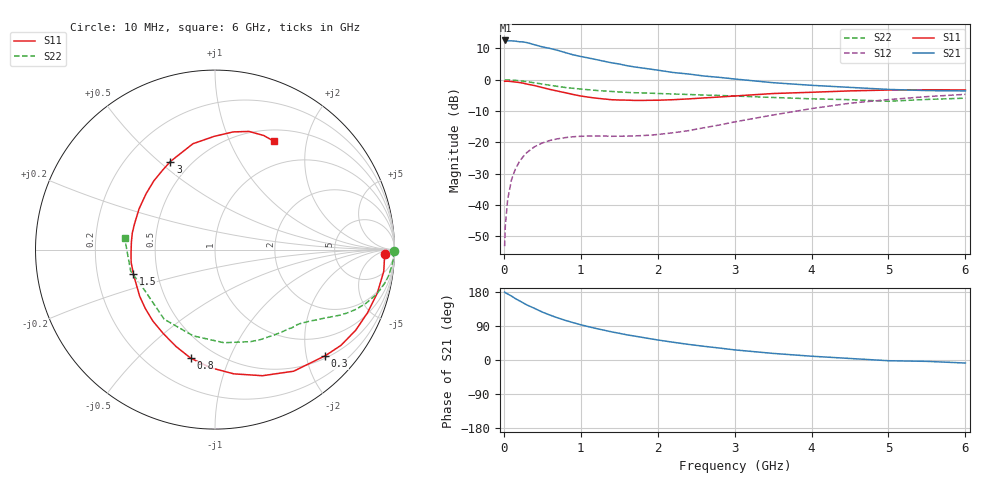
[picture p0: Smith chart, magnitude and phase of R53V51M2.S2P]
! SIEMENS Small Signal Semiconductors
! BFR183
! Si NPN RF Bipolar Junction Transistor in SOT23
! VCE = 3.5 V  IC = 1.2 mA
! Common Emitter S-Parameters:  May  1996
# GHz  S  MA  R  50
!  f  S11  S21  S12  S22
! GHz  MAG  ANG  MAG  ANG  MAG  ANG  MAG  ANG
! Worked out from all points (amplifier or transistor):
!   36 points, 10 MHz to 6 GHz, reference 50 ohm
!   highest |S21| = 12.5 dB at 20 MHz (marker M1)
!   |S21| within 3 dB of that: start of sweep to 673.1 MHz
!   unconditionally stable (mu >= 1): 1.587 GHz to 2.907 GHz
!   at 250 MHz: K = 0.17, MSG = 18.3 dB, |S12| = -24.6 dB
!   at 1.4 GHz: K = 0.90, MSG = 11.7 dB, |S12| = -18.1 dB
!   at 6 GHz: K = 0.94, MSG = 0.5 dB, |S12| = -4.7 dB
!   S11 on the Smith chart (normalised r, x): 10 MHz: 29, -15; 300 MHz: 0.55, -2.37; 800 MHz: 0.37, -0.73; 1.5 GHz: 0.36, -0.13; 3 GHz: 0.39, +0.55; 6 GHz: 0.65, +1.48
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0.01  0.9467 -1.6  4.193 179.2  0.0022 92.4  0.9976 -0.6
0.02  0.9453 -3.1  4.24 177.5  0.0048 90.3  0.9937 -1.1
0.05  0.9481 -7.3  4.185 174.2  0.0123 85.8  0.9956 -2.8
0.1  0.936 -15.1  4.178 168.6  0.0254 81.0  0.988 -5.5
0.15  0.9194 -22.6  4.136 162.0  0.0375 76.4  0.9787 -8.5
0.25  0.8818 -37.2  4.017 150.8  0.0591 68.2  0.9494 -13.3
0.3  0.8527 -43.9  3.916 145.2  0.0689 64.7  0.9315 -15.7
0.5  0.7506 -69.4  3.351 126.5  0.0979 52.4  0.8539 -22.9
0.6  0.7001 -81.4  3.161 118.5  0.1074 47.2  0.8156 -25.7
0.7  0.6584 -92.2  2.945 111.2  0.114 43.5  0.7825 -27.9
0.8  0.6198 -102.6  2.712 104.6  0.1191 39.9  0.7519 -29.8
0.9  0.5822 -111.8  2.501 98.6  0.123 37.7  0.7297 -31.3
1.1  0.5274 -131.1  2.226 88.0  0.126 34.7  0.6921 -34.4
1.3  0.4937 -148.2  1.977 78.8  0.1264 33.7  0.6613 -37.0
1.5  0.4747 -163.3  1.783 70.5  0.1255 35.0  0.6381 -39.7
1.9  0.47 168.6  1.481 56.2  0.1301 41.3  0.6109 -45.5
2.2  0.4801 151.9  1.306 46.9  0.1422 47.4  0.5922 -50.5
3  0.5502 116.9  1.028 26.7  0.2124 56.3  0.5499 -68.8
3.5  0.6025 101.8  0.897 17.4  0.2735 54.4  0.5212 -84.5
4.5  0.6636 81.2  0.755 4.0  0.4221 42.0  0.4802 -126.2
5.5  0.6913 66.8  0.671 -3.6  0.5377 25.5  0.4849 -165.7
6  0.6871 61.3  0.663 -8.0  0.5847 15.6  0.508 172.4
